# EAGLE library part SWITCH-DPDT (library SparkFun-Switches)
Double-Pole, Double-Throw (DPDT) Switch Double-pole, double-throw switches. Variant Overview PTH-GPI-152-3013 Used on SparkFun Geiger Counter SMD-AY0202 Surface Mount DPDT Switch (COM-00597) Used on e.g. LilyPad Arduino USB - ATmega32U4 Board
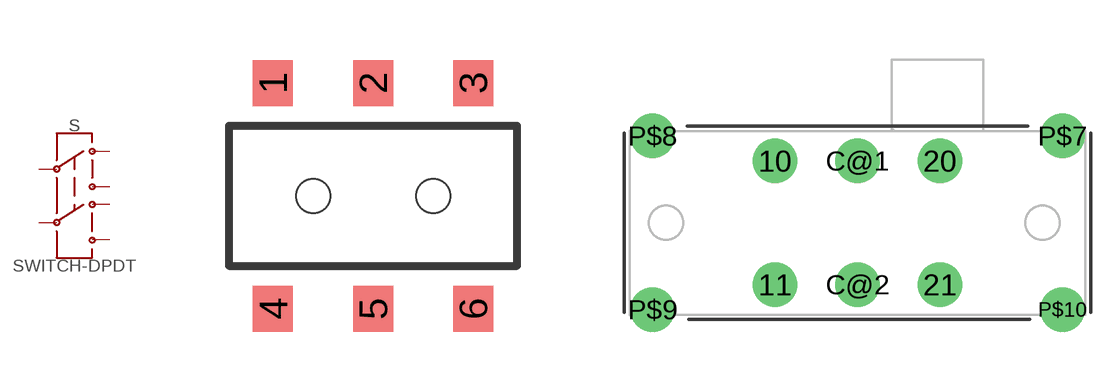
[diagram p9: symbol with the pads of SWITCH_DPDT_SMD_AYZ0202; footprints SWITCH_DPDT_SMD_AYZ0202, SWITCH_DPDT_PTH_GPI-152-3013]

Designator prefix S

## SWITCH-DPDT-SMD-AYZ0202 (PROD_ID: SWCH-08179; SF_SKU: COM-00597)  [SWITCH_DPDT_SMD_AYZ0202]
1  1
2  2
3  3
4  4
5  5
6  6

## SWITCH-DPDT-PTH-GPI-152-3013 (PROD_ID: SWCH-10554)  [SWITCH_DPDT_PTH_GPI-152-3013]
10  1
11  4
20  3
21  6
C@1  2
C@2  5

## SWITCH-DPDT-SMD-JS202011JCQN (PROD_ID: SWCH-14133)  [SWITCH_DPDT_SMD_JS202011JCQN]
1  1
2  2
3  3
4  6
5  5
6  4

## Footprint SWITCH_DPDT_SMD_AYZ0202 (pad centres in mm)
ITT Industries AYZ0202 DPDT Switch - SMD Double-pole, double-throw switches. Datasheet
smd 1 x 1.15: 1 -2.5,2.825; 2 0,2.825; 3 2.5,2.825; 4 -2.5,-2.825; 5 0,-2.825; 6 2.5,-2.825
hole 0.85 at 1.5,0
hole 0.85 at -1.5,0

## Footprint SWITCH_DPDT_PTH_GPI-152-3013 (pad centres in mm)
CW Industries GPI-152-3013 DPDT Switch - PTH Double-pole, double-throw switches. Dimensional Drawing
drill 1.65: 10 -4.6,3.455; 11 -4.6,-3.455; 20 4.6,3.455; 21 4.6,-3.455; C@1 0,3.455; C@2 0,-3.455; P$7 11.43,4.85; P$8 -11.43,4.85; P$9 -11.43,-4.85; P$10 11.43,-4.85

## Footprint SWITCH_DPDT_SMD_JS202011JCQN (pad centres in mm)
smd 1 x 1.6: 1 -2.5,-1.2; 2 0,-1.2; 3 2.5,-1.2; 4 2.5,1.2; 5 0,1.2; 6 -2.5,1.2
